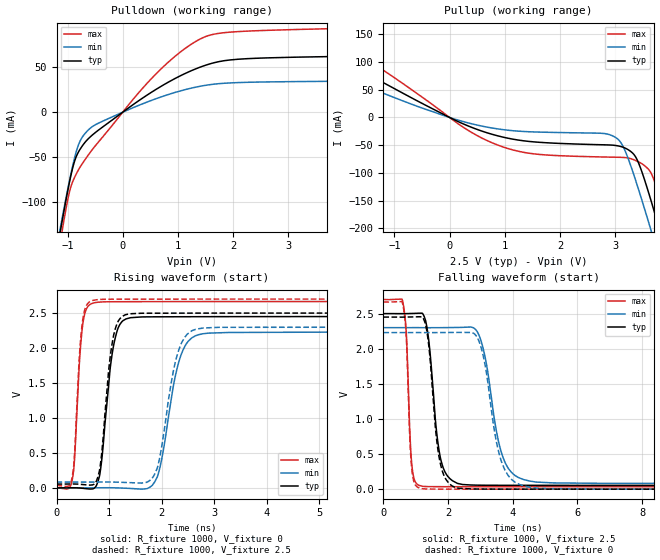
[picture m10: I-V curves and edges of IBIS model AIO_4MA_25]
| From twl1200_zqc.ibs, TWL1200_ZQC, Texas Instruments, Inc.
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[Model]   AIO_4MA_25
Model_type  Output
Vref =   2.5
Rref =   1M
Cref =   15p
Vmeas =   1.25
| variable   typ   min   max
C_comp   3.62pF   2.68pF   4.78pF
| C_pullup   3.86pF   2.68pF   4.78pF
| C_pulldown   3.38pF   2.88pF   3.93pF
[Temperature Range]   40   100   -40
| Ambient temperature   25   85   -40
[Voltage range]   2.5   2.3   2.7
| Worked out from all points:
|   slope of the pulldown table from 0 to 0.375 V, typ, clamps not added: 23.1 ohm
|   slope of the pullup table from 0 to 0.375 V, typ, clamps not added: 22.2 ohm
|   rising waveform, R_fixture 1000, V_fixture 0: 20-80 % time 196ps typ, 311ps min, 117ps max; typ from 0 V to 2.45 V
|   falling waveform, R_fixture 1000, V_fixture 2.5: 20-80 % time 296ps typ, 492ps min, 130ps max; typ from 2.5 V to 0.054 V
|   rising waveform, R_fixture 1000, V_fixture 2.5: 20-80 % time 181ps typ, 294ps min, 115ps max; typ from 0.054 V to 2.5 V
|   falling waveform, R_fixture 1000, V_fixture 0: 20-80 % time 288ps typ, 477ps min, 127ps max; typ from 2.45 V to 0 V
[Pulldown]
| AIO_4MA_25
|   Voltage   I(typ)   I(min)   I(max)
-2.5V     -646.8mA   -614mA     -695.8mA
-1.145V   -137.1mA   -132.8mA   -149.3mA
-1.105V   -123.1mA   -119.6mA   -134.3mA
-1.08V    -114.6mA   -111.5mA   -125.1mA
-960mV    -76.07mA   -74.26mA   -87.05mA
-875mV    -54.83mA   -51.19mA   -72.56mA
-775mV    -41.29mA   -32.28mA   -61.08mA
-625mV    -29.5mA    -19.8mA    -47.56mA
570mV     23.99mA    14.19mA    40.37mA
1.405V    49.97mA    28.75mA    81.18mA
2.24V     59.27mA    33.09mA    89.82mA
5V        62.72mA    34.67mA    94.24mA
[Pullup]
| AIO_4MA_25
|   Voltage   I(typ)   I(min)   I(max)
-2.5V     130mA      93.97mA    163.5mA
-430mV    21.91mA    14.65mA    31.96mA
770mV     -30.37mA   -19.01mA   -45.69mA
1.535V    -44.12mA   -26.1mA    -65.78mA
2.94V     -49.87mA   -32.57mA   -71.64mA
3.125V    -53.09mA   -48.77mA   -72.04mA
3.345V    -67.36mA   -105.4mA   -76.58mA
3.47V     -93.89mA   -144.5mA   -82.6mA
3.64V     -146.7mA   -200.3mA   -98.43mA
3.795V    -199.4mA   -252.6mA   -141.3mA
3.95V     -254mA     -305.7mA   -196.1mA
5V        -640.1mA   -677.1mA   -599.8mA
[Ramp]
| AIO_4MA_25
| variable   typ   min   max
dV/dt_r   1.48/2.16E-10   1.35/3.16E-10   1.61/1.24E-10
dV/dt_f   1.47/3.06E-10   1.34/5.00E-10   1.60/1.31E-10
R_load = 1000
[Rising Waveform]
| AIO_4MA_25
R_fixture =   1000
C_fixture =   0
L_fixture =   0
V_fixture =   0
V_fixture_min = 0
V_fixture_max = 0
|   Time   V(typ)   V(min)   V(max)
0s        9.669nV    39.64nV    988pV
310ps     1.509mV    -21.23uV   162.8mV
535ps     -9.333mV   -43.86uV   2.482V
815ps     158mV      1.198mV    2.656V
975ps     1.327V     1.817mV    2.661V
1.27ns    2.393V     -3.574mV   2.662V
1.92ns    2.446V     157.5mV    2.663V
2.475ns   2.447V     2.063V     2.664V
3.28ns    2.449V     2.222V     2.664V
238.2ns   2.45V      2.23V      2.665V
[Falling Waveform]
| AIO_4MA_25
R_fixture =   1000
C_fixture =   0
L_fixture =   0
V_fixture =   2.5
V_fixture_min = 2.3
V_fixture_max = 2.7
|   Time   V(typ)   V(min)   V(max)
0s        2.5V       2.3V       2.7V
590ps     2.499V     2.3V       2.686V
900ps     2.502V     2.3V       263.1mV
1.37ns    2.233V     2.299V     36.64mV
1.69ns    646.4mV    2.3V       35.59mV
1.99ns    182.8mV    2.301V     35.25mV
2.955ns   56.7mV     2.194V     34.65mV
3.87ns    54.82mV    290.7mV    34.45mV
5.275ns   54.27mV    88.96mV    34.32mV
238.2ns   54mV       82.44mV    34.26mV
[Rising Waveform]
| AIO_4MA_25
R_fixture =   1000
C_fixture =   0
L_fixture =   0
V_fixture =   2.5
V_fixture_min = 2.3
V_fixture_max = 2.7
|   Time   V(typ)   V(min)   V(max)
0s        54mV       82.44mV    34.26mV
285ps     55.41mV    82.42mV    106mV
495ps     47.59mV    82.4mV     2.382V
760ps     97.66mV    83.11mV    2.689V
970ps     1.475V     83.79mV    2.698V
1.25ns    2.452V     78.77mV    2.699V
1.895ns   2.498V     238mV      2.699V
2.435ns   2.499V     2.145V     2.699V
3.105ns   2.499V     2.296V     2.7V
238.2ns   2.5V       2.3V       2.7V
[Falling Waveform]
| AIO_4MA_25
R_fixture =   1000
C_fixture =   0
L_fixture =   0
V_fixture =   0
V_fixture_min = 0
V_fixture_max = 0
|   Time   V(typ)   V(min)   V(max)
0s        2.45V      2.23V      2.665V
590ps     2.45V      2.23V      2.65V
700ps     2.45V      2.23V      2.229V
895ps     2.453V     2.23V      219.5mV
1.335ns   2.273V     2.229V     2.543mV
1.805ns   283.7mV    2.23V      1.032mV
2.725ns   3.33mV     2.231V     442.2uV
3.76ns    753.3uV    269.7mV    192.7uV
5.17ns    255uV      6.101mV    69.59uV
238.2ns   43.88nV    92.26nV    17.03nV
